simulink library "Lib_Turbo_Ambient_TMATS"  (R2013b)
settings: Solver=ode45  StartTime=0.0  StopTime=10.0  RelTol=1e-3

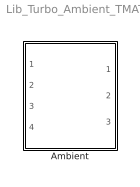
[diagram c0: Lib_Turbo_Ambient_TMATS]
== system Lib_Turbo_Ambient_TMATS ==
  Ambient : Subsystem

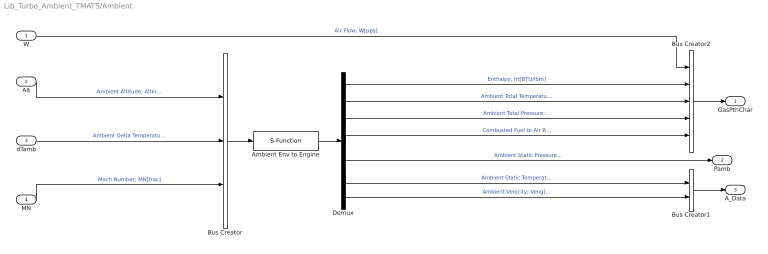
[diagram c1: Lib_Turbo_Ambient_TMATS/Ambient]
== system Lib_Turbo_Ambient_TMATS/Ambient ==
  W : Inport
  Alt : Inport  Port=2
  dTamb : Inport  Port=3
  MN : Inport  Port=4
  Ambient Env to Engine : S-Function  FunctionName=Ambient_TMATS  Parameters="X_A_AltVec_M, T_A_TsVec_M, T_A_PsVec_M, X_A_FARVec_M, Y_A_TVec_M, T_A_RtArray_M, T_A_gammaArray_M, AFARc_M,   gcs"  EnableBusSupport=off
  Bus Creator : BusCreator  Inputs=3
  Bus Creator1 : BusCreator  Inputs=2
  Bus Creator2 : BusCreator  Inputs=5
  Demux : Demux  Outputs=7
  GasPthChar : Outport
  Pamb : Outport  Port=2
  A_Data : Outport  Port=3
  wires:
  Demux/6 -> Bus Creator1/1  "Ambient Static Temperature; Ts[degR]"
  Demux/5 -> Pamb/1  "Ambient Static Pressure; Ps[psia]"
  Ambient Env to Engine/1 -> Demux/1
  Demux/2 -> Bus Creator2/3  "Ambient Total Temperature; Tt[degR]"
  Demux/3 -> Bus Creator2/4  "Ambient Total Pressure; Pt [psia]"
  Bus Creator/1 -> Ambient Env to Engine/1
  dTamb/1 -> Bus Creator/2  "Ambient Delta Temperature; dTambIn[degF]"
  MN/1 -> Bus Creator/3  "Mach Number; MN[frac]"
  Alt/1 -> Bus Creator/1  "Ambient Altitude; AltIn[ft]"
  Demux/7 -> Bus Creator1/2  "Ambient Velocity; Veng[ft/sec]"
  Demux/4 -> Bus Creator2/5  "Combusted Fuel to Air Ratio; FARc [frac]"
  Bus Creator1/1 -> A_Data/1
  Demux/1 -> Bus Creator2/2  "Enthalpy; ht[BTU/lbm]"
  W/1 -> Bus Creator2/1  "Air Flow; W[pps]"
  Bus Creator2/1 -> GasPthChar/1
